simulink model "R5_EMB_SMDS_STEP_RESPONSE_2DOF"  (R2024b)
settings: Solver=ode5  StartTime=0.0  StopTime=S  FixedStep=T  RelTol=1e-3  EnableMultiTasking=on
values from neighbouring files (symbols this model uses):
  Kt = Kt*motor_eff    (= 0.0273)    [R5_EMB_SMDS_STEP_RESPONESE_2DOF_script.m]
  r = 0.01    [R5_EMB_SMDS_STEP_RESPONESE_2DOF_script.m]
  T = 0.002    [R5_EMB_SMDS_STEP_RESPONESE_2DOF_script.m]
undefined symbols (not defined in the file or in its folder): Serial_Port, Standard_Devices
libraries: easyio x7, simulink x3

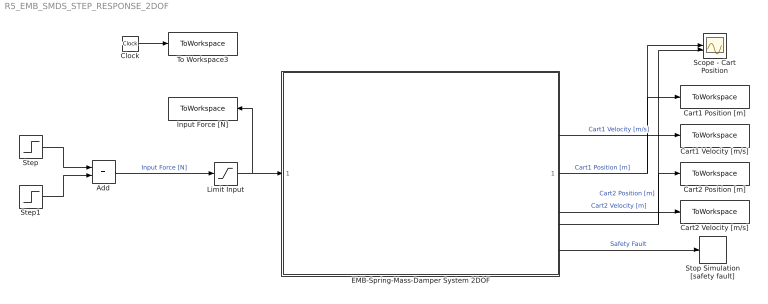
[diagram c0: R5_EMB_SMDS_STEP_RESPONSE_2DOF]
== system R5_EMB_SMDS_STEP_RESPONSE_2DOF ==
  Add : Sum
  Cart1 Position [m] : ToWorkspace  VariableName=cart1_position  SampleTime=T
  Cart1 Velocity [m/s] : ToWorkspace  VariableName=cart1_velocity  SampleTime=T
  Cart2 Position [m] : ToWorkspace  VariableName=cart2_position  SampleTime=T
  Cart2 Velocity [m/s] : ToWorkspace  VariableName=cart2_velocity  SampleTime=T
  Clock : Clock
  EMB-Spring-Mass-Damper System 2DOF : Subsystem
  Input Force [N] : ToWorkspace  VariableName=f_input  SampleTime=T
  Limit Input : Saturate  UpperLimit=10  LowerLimit=-10
  Scope - Cart Position : Scope  NumInputPorts=2
  Step : Step  After=3  SampleTime=T
  Step1 : Step  Time=2  After=-3  SampleTime=T
  Stop Simulation [safety fault] : Stop
  To Workspace3 : ToWorkspace  VariableName=rt_time  SampleTime=T
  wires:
  Clock/1 -> To Workspace3/1
  EMB-Spring-Mass-Damper System 2DOF/1(Out1) -> Scope - Cart Position/1, Cart1 Position [m]/1  "Cart1 Position [m]"
  EMB-Spring-Mass-Damper System 2DOF/5(Out5) -> Stop Simulation [safety fault]/1  "Safety Fault"
  EMB-Spring-Mass-Damper System 2DOF/2(Out2) -> Cart1 Velocity [m/s]/1  "Cart1 Velocity [m/s]"
  Limit Input/1 -> EMB-Spring-Mass-Damper System 2DOF/1(In1), Input Force [N]/1
  Add/1 -> Limit Input/1  "Input Force [N]"
  Step/1 -> Add/1
  Step1/1 -> Add/2
  EMB-Spring-Mass-Damper System 2DOF/3(Out3) -> Scope - Cart Position/2, Cart2 Position [m]/1  "Cart2 Position [m]"
  EMB-Spring-Mass-Damper System 2DOF/4(Out4) -> Cart2 Velocity [m/s]/1  "Cart2 Velocity [m]"

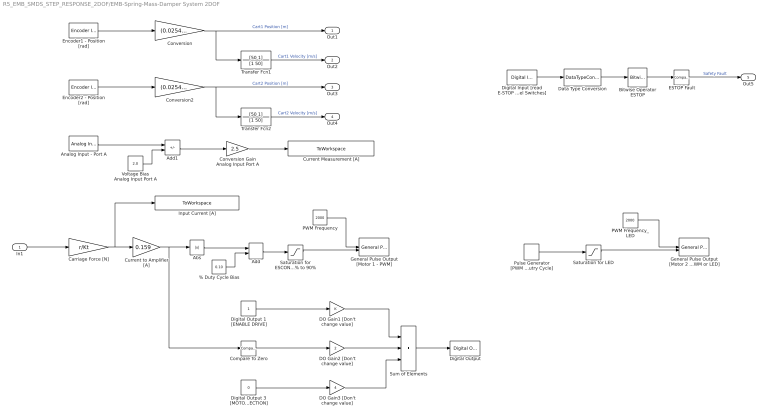
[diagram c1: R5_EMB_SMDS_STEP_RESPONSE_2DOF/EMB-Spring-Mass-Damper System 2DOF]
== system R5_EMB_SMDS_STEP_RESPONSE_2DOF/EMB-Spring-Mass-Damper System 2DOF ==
  In1 : Inport
  % Duty Cycle Bias : Constant  Value=0.10  SampleTime=T
  Abs : Abs
  Add : Sum
  Add1 : Sum  Inputs=+-
  Analog Input - Port A : easyio/Analog Input  SampleTime=T  MaxMissedTicks=10  ShowMissedTicks=0  YieldWhenWaiting=0  DrvName=Standard_Devices/Serial_Port  DrvAddress=6  DrvOptions=[460800 8 0 0 0 0 0 0]  PacketSize=8  DataTypes='double'  ShowReady=0  ShowError=0  PacketID=1  ByteOrder=1  ShowTimestamp=0  CfgPrm=A6  PrmCfg=unipolar  ResVar=0  VarRes=0
  Bitwise Operator ESTOP : simulink/Logic and Bit Operations/Bitwise Operator  logicop=AND  UseBitMask=on  BitMask=8  BitMaskRealWorld=Real World Value
  Carriage Force [N] : Gain  Gain=r/Kt
  Compare To Zero : simulink/Logic and Bit Operations/Compare To Zero  relop=>=  OutDataTypeStr=boolean
  Conversion : Gain  Gain=(0.0254)/(2*pi)
  Conversion Gain Analog Input Port A : Gain  Gain=2.5
  Conversion2 : Gain  Gain=(0.0254)/(2*pi)
  Current Measurement [A] : ToWorkspace  VariableName=i_measure  SampleTime=T
  Current to Amplifier [A] : Gain  Gain=0.159
  DO Gain1 [Don't change value] : Gain
  DO Gain2 [Don't change value] : Gain  Gain=2
  DO Gain3 [Don't change value] : Gain  Gain=4
  Data Type Conversion : DataTypeConversion  OutDataTypeStr=uint8  RndMeth=Nearest
  Digital Input [read E-STOP and End of Travel Switches] : easyio/Digital Input  SampleTime=T  MaxMissedTicks=10  ShowMissedTicks=0  YieldWhenWaiting=0  DrvName=Standard_Devices/Serial_Port  DrvAddress=6  DrvOptions=[460800 8 0 0 0 0 0 0]  PacketSize=8  DataTypes='double'  ShowReady=0  ShowError=0  PacketID=1  ByteOrder=1  ShowTimestamp=0  CfgPrm=D0  PrmCfg=18  ResVar=0  VarRes=0  d7=off  d6=off  d5=off  d4=on  d3=on  d2=off  d1=off  d0=off
  Digital Output : easyio/Digital Output  SampleTime=T  MaxMissedTicks=10  ShowMissedTicks=0  YieldWhenWaiting=0  DrvName=Standard_Devices/Serial_Port  DrvAddress=6  DrvOptions=[460800 8 0 0 0 0 0 0]  PacketSize=8  DataTypes='double'  ShowReady=0  ShowError=0  PacketID=1  ByteOrder=1  InitialValue=0  FinalValue=0  CfgPrm=G0  PrmCfg=F8  ResVar=0  VarRes=0  d7=off  d6=off  d5=off  d4=off  d3=off  d2=on  d1=on  d0=on
  Digital Output 1 [ENABLE DRIVE] : Constant  SampleTime=T
  Digital Output 3 [MOTOR 2 DIRECTION] : Constant  Value=0  SampleTime=T
  ESTOP Fault : simulink/Logic and Bit Operations/Compare To Constant  relop=~=  const=8  OutDataTypeStr=boolean
  Encoder1 - Position [rad] : easyio/Encoder Input  SampleTime=T  MaxMissedTicks=10  ShowMissedTicks=0  YieldWhenWaiting=0  DrvName=Standard_Devices/Serial_Port  DrvAddress=6  DrvOptions=[460800 8 0 0 0 0 0 0]  PacketSize=8  DataTypes='double'  ShowReady=0  ShowError=0  PacketID=1  ByteOrder=1  ShowTimestamp=0  CfgPrm=E0  PrmCfg=position  ResVar=0  VarRes=2000
  Encoder2 - Position [rad] : easyio/Encoder Input  SampleTime=T  MaxMissedTicks=10  ShowMissedTicks=0  YieldWhenWaiting=0  DrvName=Standard_Devices/Serial_Port  DrvAddress=6  DrvOptions=[460800 8 0 0 0 0 0 0]  PacketSize=8  DataTypes='double'  ShowReady=0  ShowError=0  PacketID=1  ByteOrder=1  ShowTimestamp=0  CfgPrm=E1  PrmCfg=position  ResVar=0  VarRes=2000
  General Pulse Output [Motor 1 - PWM] : easyio/General Pulse Output  SampleTime=T  MaxMissedTicks=10  ShowMissedTicks=0  YieldWhenWaiting=0  DrvName=Standard_Devices/Serial_Port  DrvAddress=6  DrvOptions=[460800 8 0 0 0 0 0 0]  PacketSize=16  DataTypes={'double','double'}  ShowReady=0  ShowError=0  PacketID=1  ByteOrder=1  InitialValue=[0 0]  FinalValue=[0 0]  CfgPrm=N0  PrmCfg=frequency and duty  ResVar=449.8360 Hz - 115156.25 Hz  VarRes=64
  General Pulse Output [Motor 2 - PWM or LED] : easyio/General Pulse Output  SampleTime=T  MaxMissedTicks=10  ShowMissedTicks=0  YieldWhenWaiting=0  DrvName=Standard_Devices/Serial_Port  DrvAddress=6  DrvOptions=[460800 8 0 0 0 0 0 0]  PacketSize=16  DataTypes={'double','double'}  ShowReady=0  ShowError=0  PacketID=1  ByteOrder=1  InitialValue=[0 0]  FinalValue=[0 0]  CfgPrm=N1  PrmCfg=frequency and duty  ResVar=449.8360 Hz - 115156.25 Hz  VarRes=64
  Input Current [A] : ToWorkspace  VariableName=i_input  SampleTime=T
  PWM Frequency : Constant  Value=2000  SampleTime=T
  PWM Frequency_LED : Constant  Value=2000  SampleTime=T
  Pulse Generator [PWM % Dutry Cycle] : DiscretePulseGenerator  PulseType=Time based  Period=0.4  PulseWidth=50
  Saturation for ESCON 10% to 90% : Saturate  UpperLimit=0.9  LowerLimit=0.1
  Saturation for LED : Saturate  UpperLimit=1  LowerLimit=0
  Sum of Elements : Sum  Inputs=+++
  Transfer Fcn1 : TransferFcn  Numerator=[50 1]  Denominator=[1 50]
  Transfer Fcn2 : TransferFcn  Numerator=[50 1]  Denominator=[1 50]
  Voltage Bias Analog Input Port A : Constant  Value=2.0
  Out1 : Outport
  Out2 : Outport  Port=2
  Out3 : Outport  Port=3
  Out4 : Outport  Port=4
  Out5 : Outport  Port=5
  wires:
  ESTOP Fault/1 -> Out5/1  "Safety Fault"
  % Duty Cycle Bias/1 -> Add/2
  Conversion Gain Analog Input Port A/1 -> Current Measurement [A]/1
  Add1/1 -> Conversion Gain Analog Input Port A/1
  Current to Amplifier [A]/1 -> Abs/1, Compare To Zero/1
  Saturation for ESCON 10% to 90%/1 -> General Pulse Output [Motor 1 - PWM]/2
  Voltage Bias Analog Input Port A/1 -> Add1/2
  DO Gain2 [Don't change value]/1 -> Sum of Elements/2
  Analog Input - Port A/1 -> Add1/1
  PWM Frequency/1 -> General Pulse Output [Motor 1 - PWM]/1
  Conversion/1 -> Out1/1, Transfer Fcn1/1  "Cart1 Position [m]"
  DO Gain1 [Don't change value]/1 -> Sum of Elements/1
  Digital Output 1 [ENABLE DRIVE]/1 -> DO Gain1 [Don't change value]/1
  Saturation for LED/1 -> General Pulse Output [Motor 2 - PWM or LED]/2
  PWM Frequency_LED/1 -> General Pulse Output [Motor 2 - PWM or LED]/1
  Carriage Force [N]/1 -> Input Current [A]/1, Current to Amplifier [A]/1
  Pulse Generator [PWM % Dutry Cycle]/1 -> Saturation for LED/1
  Encoder1 - Position [rad]/1 -> Conversion/1
  Sum of Elements/1 -> Digital Output/1
  Add/1 -> Saturation for ESCON 10% to 90%/1
  Compare To Zero/1 -> DO Gain2 [Don't change value]/1
  Abs/1 -> Add/1
  In1/1 -> Carriage Force [N]/1
  Digital Output 3 [MOTOR 2 DIRECTION]/1 -> DO Gain3 [Don't change value]/1
  DO Gain3 [Don't change value]/1 -> Sum of Elements/3
  Transfer Fcn1/1 -> Out2/1  "Cart1 Velocity [m/s]"
  Bitwise Operator ESTOP/1 -> ESTOP Fault/1
  Data Type Conversion/1 -> Bitwise Operator ESTOP/1
  Digital Input [read E-STOP and End of Travel Switches]/1 -> Data Type Conversion/1
  Transfer Fcn2/1 -> Out4/1  "Cart2 Velocity [m/s]"
  Encoder2 - Position [rad]/1 -> Conversion2/1
  Conversion2/1 -> Transfer Fcn2/1, Out3/1  "Cart2 Position [m]"
